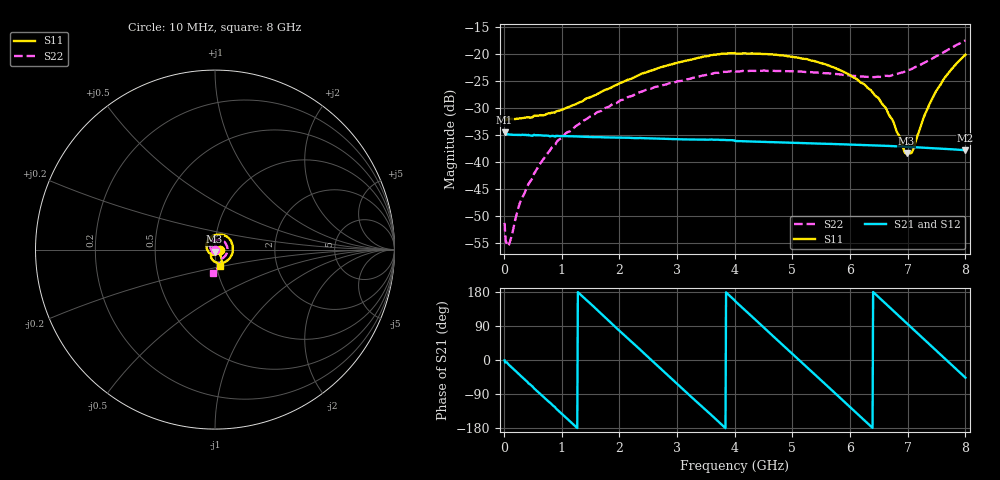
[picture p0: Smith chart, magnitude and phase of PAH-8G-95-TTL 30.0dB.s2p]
! MTS Systemtechnik GmbH
! S-Parameters
! Model: PAH-8G/95-TTL
! Attenuation Step: 30.0dB
! Rohde & Schwarz ZVB8 2Ports - Version 4.11 - 1145.1010k08 SN: 100119
! S2P File Measurements:
! S11 S21 S12 S22
# HZ  S  DB  R  50.00
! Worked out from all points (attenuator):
!   800 points, 10 MHz to 8 GHz, reference 50 ohm
!   highest |S21| = -34.49 dB at 10 MHz (marker M1); lowest = -37.8 dB at 8 GHz (marker M2)
!   lowest |S11| = -38.4 dB at 6.98 GHz (marker M3), VSWR 1.02, Z = 49.7 - j1.17 ohm
!   |S11| at or under -10 dB: start of sweep to end of sweep
!   |S22| runs from -55.5 to -17.6 dB; largest |S21 - S12| = 0.00028
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1e7  -31.74 -5.3  -34.49 -1.2  -34.40 -1.1  -51.21 -124.5
6e7  -32.12 -6.8  -34.86 -8.3  -34.87 -8.2  -55.41 -144.8
9e7  -32.05 -10.8  -34.90 -13.4  -34.89 -13.4  -55.13 -132.2
2.8e8  -31.94 -31.2  -34.99 -40.4  -34.99 -40.4  -47.39 -121.6
5.6e8  -31.45 -62.8  -35.02 -80.4  -35.05 -80.1  -41.43 -138.9
9.4e8  -30.55 -105.5  -35.18 -133.3  -35.16 -133.3  -35.96 -163.8
1.35e9  -28.82 -149.0  -35.31 169.2  -35.31 169.2  -32.59 169.7
2.02e9  -25.38 153.5  -35.49 74.7  -35.50 74.9  -28.59 129.4
2.68e9  -22.63 107.4  -35.67 -18.0  -35.67 -17.7  -26.03 94.9
3.43e9  -20.63 60.8  -35.84 -122.5  -35.85 -122.6  -24.07 57.2
4.01e9  -19.98 24.5  -36.11 155.0  -36.10 154.9  -23.30 28.4
4.65e9  -20.15 -14.5  -36.32 65.1  -36.33 65.0  -23.14 -1.0
5.34e9  -21.28 -56.9  -36.54 -31.4  -36.54 -31.4  -23.42 -30.5
6.11e9  -24.64 -104.5  -36.80 -139.9  -36.82 -139.8  -24.13 -55.7
6.49e9  -28.18 -126.0  -36.95 166.8  -36.95 166.6  -24.24 -62.5
6.67e9  -31.18 -131.2  -37.02 141.3  -37.02 141.3  -24.13 -64.4
6.98e9  -38.40 -102.6  -37.18 97.4  -37.18 97.4  -23.12 -68.1
7.09e9  -37.79 -64.6  -37.23 81.9  -37.24 81.9  -22.69 -69.6
7.29e9  -31.42 -43.0  -37.34 53.7  -37.34 53.6  -21.66 -72.7
7.5e9  -26.78 -46.6  -37.46 24.0  -37.46 24.0  -20.44 -77.4
7.72e9  -23.38 -57.3  -37.61 -7.0  -37.61 -7.1  -19.14 -84.4
8e9  -20.19 -73.5  -37.82 -46.6  -37.82 -46.5  -17.56 -95.2
